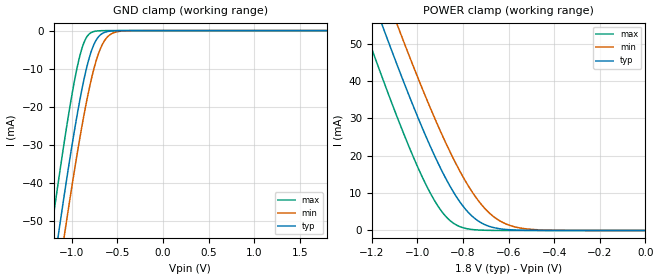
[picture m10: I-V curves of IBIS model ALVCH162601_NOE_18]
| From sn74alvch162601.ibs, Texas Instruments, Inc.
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[Model]   ALVCH162601_NOE_18
Model_type  Input
Vinl=0.5775
Vinh=1.2675
| variable   typ   min   max
C_comp   2.01pF   1.69pF   2.23pF
[Temperature Range]   40   100   -40
| Ambient temperature   25   85   -40
[Voltage range]   1.8   1.65   1.95
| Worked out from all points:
|   GND clamp passes 1 mA (typ) near -0.68 V on its own axis
|   POWER clamp passes 1 mA (typ) near -0.68 V on its own axis
[GND Clamp]
| ALVCH162601_NOE_18
|   Voltage   I(typ)   I(min)   I(max)
-1.8V     -169.5mA   -179.7mA   -156.7mA
-1.245V   -70.18mA   -81.02mA   -56.25mA
-1.22V    -65.92mA   -76.78mA   -51.96mA
-1.14V    -52.55mA   -63.42mA   -38.55mA
-1.075V   -42.06mA   -52.87mA   -28.16mA
-920mV    -19.37mA   -29.44mA   -7.486mA
-860mV    -12.16mA   -21.41mA   -2.808mA
-795mV    -6.112mA   -13.8mA    -645.2uA
-730mV    -2.404mA   -7.745mA   -117.8uA
-660mV    -692.8uA   -3.429mA   -17.66uA
-495mV    -25.94uA   -271uA     -195.5nA
1.8V      1.111nA    770.5nA    2.881pA
[POWER Clamp]
| ALVCH162601_NOE_18
|   Voltage   I(typ)   I(min)   I(max)
-1.8V     169.5mA    179.7mA    156.7mA
-1.235V   68.47mA    79.32mA    54.53mA
-1.155V   55.02mA    65.9mA     41.02mA
-1.135V   51.73mA    62.6mA     37.73mA
-1.08V    42.85mA    53.67mA    28.94mA
-930mV    20.68mA    30.85mA    8.514mA
-875mV    13.84mA    23.34mA    3.72mA
-825mV    8.636mA    17.15mA    1.329mA
-765mV    4.1mA      10.78mA    298.6uA
-705mV    1.577mA    5.93mA     59.98uA
-595mV    194.7uA    1.357mA    2.999uA
-16.28fV  1.111nA    59.61nA    3.661pA
